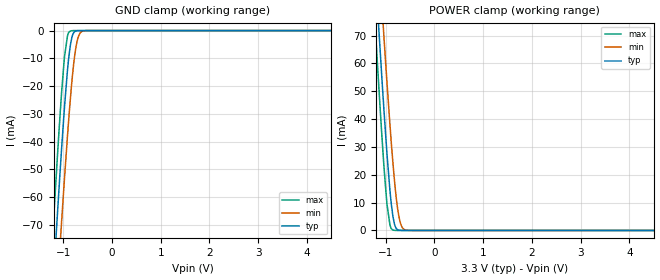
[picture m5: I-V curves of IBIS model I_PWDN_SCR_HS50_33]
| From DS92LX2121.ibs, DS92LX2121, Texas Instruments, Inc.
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|   Model I_PWDN_SCR_HS50_33
[Model] I_PWDN_SCR_HS50_33
Model_type Input
Vinl =   0.8
Vinh =   2.0
|   typ   min   max
|   (nom)   (fast)   (slow)
C_comp   0.3665pF   0.3665pF   0.5298pF
[Temperature Range]   25.000   105.000   -40.000
[Voltage Range]   3.300V   3.0000V   3.6000V
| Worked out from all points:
|   GND clamp passes 1 mA (typ) near -0.79 V on its own axis
|   POWER clamp passes 1 mA (typ) near -0.79 V on its own axis
[GND Clamp]
|   Voltage   I(typ)   I(min)   I(max)
-3.3V     -740.6mA   -745.8mA   -738.2mA
-1.211V   -92.27mA   -118mA     -71.83mA
-1.191V   -86.5mA    -112.3mA   -65.95mA
-1.112V   -63.85mA   -90.11mA   -43.04mA
-1.043V   -44.84mA   -71.14mA   -24.45mA
-973.5mV  -27.25mA   -52.87mA   -9.257mA
-914.1mV  -14.38mA   -38.09mA   -1.938mA
-854.7mV  -5.279mA   -24.66mA   -158.3uA
-785.4mV  -769.6uA   -11.9mA    -11.81uA
-726mV    -91.41uA   -4.691mA   -6.467uA
-577.5mV  -3.449uA   -99.25uA   -4.919uA
6.59V     0A         0A         0A
[POWER Clamp]
|   Voltage   I(typ)   I(min)   I(max)
-3.3V     739mA      744.2mA    736.5mA
-1.211V   92.02mA    117.6mA    71.62mA
-1.191V   86.27mA    112mA      65.75mA
-1.112V   63.66mA    89.86mA    42.89mA
-1.043V   44.7mA     70.93mA    24.36mA
-973.5mV  27.14mA    52.7mA     9.21mA
-914.1mV  14.31mA    37.95mA    1.931mA
-854.7mV  5.248mA    24.55mA    164.4uA
-785.4mV  767.3uA    11.83mA    19.72uA
-726mV    94.5uA     4.66mA     14.93uA
-577.5mV  8.162uA    100.4uA    14.65uA
6.59V     0A         0A         0A
